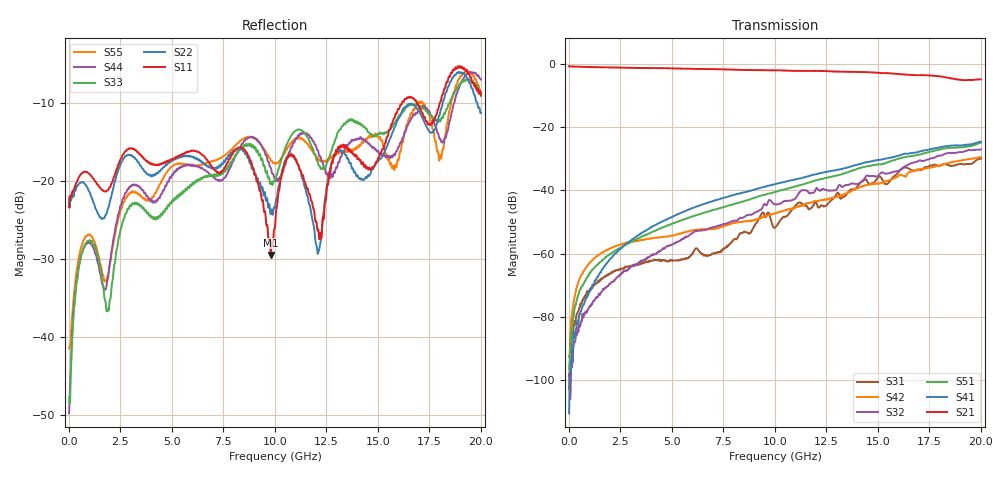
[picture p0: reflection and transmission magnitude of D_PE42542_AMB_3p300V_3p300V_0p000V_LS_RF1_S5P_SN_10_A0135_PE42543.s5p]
! Device ID: PE42542
! Device ID: PE42542
! File Path: z:\PE42542\PE42543_20140723_inv\AMB\3p300\LS_RF1\PE42542_AMB_3p300V_3p300V_0p000V_LS_RF1_S5P_SN_10_A0135_PE42543.s5p
! Serial: 10
! Lot: A0135_PE42543
! Temp: AMB
! VDD: 3.300
! VSS: 0.000
! Control_Hi: 3.300
! Control_Lo: 0.000
! Logic State: LS_RF1
! Port 1: RFC
! Port 2: RF1
! Port 3: RF2
! Port 5: RF3
! Port 6: RF4
! ThroughPath:1-2
! IDD: -0.000136633224
! ISS: 1.33568146e-009
#  Hz  S  RI  R  50
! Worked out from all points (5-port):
!   801 points, 10 MHz to 20 GHz, reference 50 ohm
!   strongest paths, dB at 10 MHz, 5.008 GHz, 10.01 GHz, 15 GHz, 20 GHz:
!     S21: -0.7, -1.4, -2.0, -2.8, -4.9
!     S41: -110.5, -48.4, -38.0, -30.4, -24.6
!     S51: -96.5, -50.5, -40.5, -31.8, -24.9
!     S32: -98.7, -57.1, -44.3, -35.4, -27.0
!     S42: -92.4, -54.3, -47.2, -37.8, -29.4
!     S31: -102.9, -62.2, -51.7, -35.9, -29.9
!   lowest |S11| = -29.4 dB at 9.805 GHz (marker M1), VSWR 1.07, Z = 47.8 + j2.43 ohm
!   |S11| at or under -10 dB: start of sweep to 16.17 GHz; 16.89 GHz to 18 GHz (1.111 GHz wide, 6.37 % of centre)
